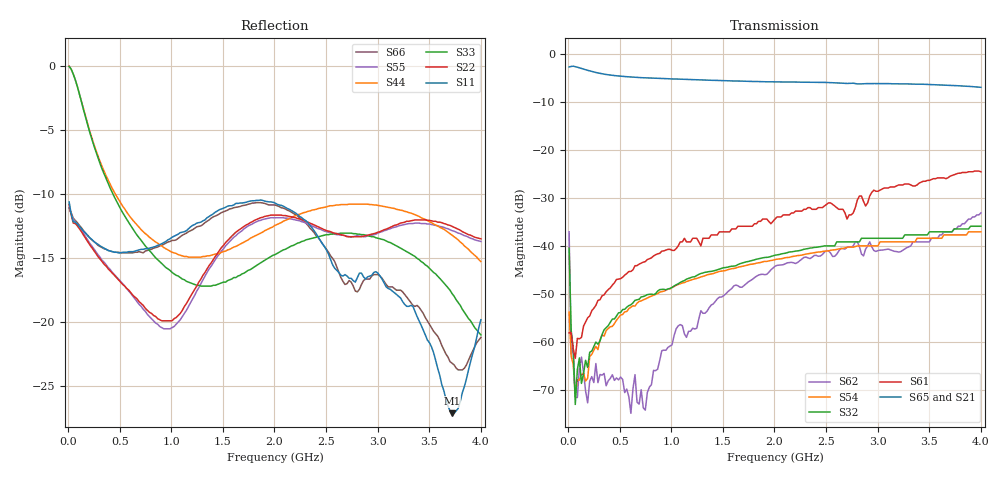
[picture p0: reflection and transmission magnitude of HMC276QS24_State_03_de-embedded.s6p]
! Hittite Microwave Corporation
! 20 Alpha Road
! Chelmsford, MA 01824
! Tel: 978-250-3343
! Fax: 978-250-3373
! Device: HMC276QS24, 0.7-3.0 GHz, GaAS MMIC 4x2 Switch Matrix in 24-lead QSOP package
! Misc: Data was de-embedded to package pins.
!  Port 1 = OP1
!  Port 2 = VL
!  Port 3 = VH
!  Port 4 = HH
!  Port 5 = HL
!  Port 6 = OP2
!  Vdd = +5 V
!  Vctl = 0 V[Logic 0] / +5 V[Logic 1]
!  State 03,  VL to OP1,  HL to OP2
!  Control Lines (Logic)
!  HV 1 = 0, Tone 1 = 0
!  HV 2 = 1, Tone 2 = 0
!  Data reformated to new Touchstone file format - Wed Jan 10 14:24:32 2007
# MHz S DB R 50
! 6 Port Network Data
! freq  dbS11  angS11  dbS12  angS12  dbS13  angS13  dbS14  angS14
!  dbS15  angS15  dbS16  angS16
!  dbS21  angS21  dbS22  angS22
!  dbS23  angS23  dbS24  angS24  dbS25  angS25  dbS26  angS26
!  dbS31  angS31  dbS32  angS32  dbS33  angS33  dbS34  angS34
!  dbS35  angS35  dbS36  angS36
!  dbS41  angS41  dbS42  angS42
!  dbS43  angS43  dbS44  angS44  dbS45  angS45  dbS46  angS46
!  dbS51  angS51  dbS52  angS52  dbS53  angS53  dbS54  angS54
!  dbS55  angS55  dbS56  angS56
!  dbS61  angS61  dbS62  angS62
!  dbS63  angS63  dbS64  angS64  dbS65  angS65  dbS66  angS66
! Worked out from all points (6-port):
!   201 points, 10 MHz to 4 GHz, reference 50 ohm
!   strongest paths, dB at 10 MHz, 1.008 GHz, 2.005 GHz, 3.002 GHz, 4 GHz:
!     S65: -2.8, -5.3, -5.9, -6.2, -7.0
!     S21: -2.9, -5.3, -5.9, -6.3, -7.1
!     S61: -58.1, -40.9, -34.4, -28.6, -24.6
!     S32: -40.5, -48.7, -41.9, -38.4, -35.9
!     S54: -53.8, -48.6, -42.9, -40.0, -37.1
!     S62: -37.1, -60.6, -44.2, -41.0, -33.2
!   lowest |S11| = -27.1 dB at 3.721 GHz (marker M1), VSWR 1.09, Z = 48.9 + j4.22 ohm
!   |S11| at or under -10 dB: start of sweep to end of sweep
